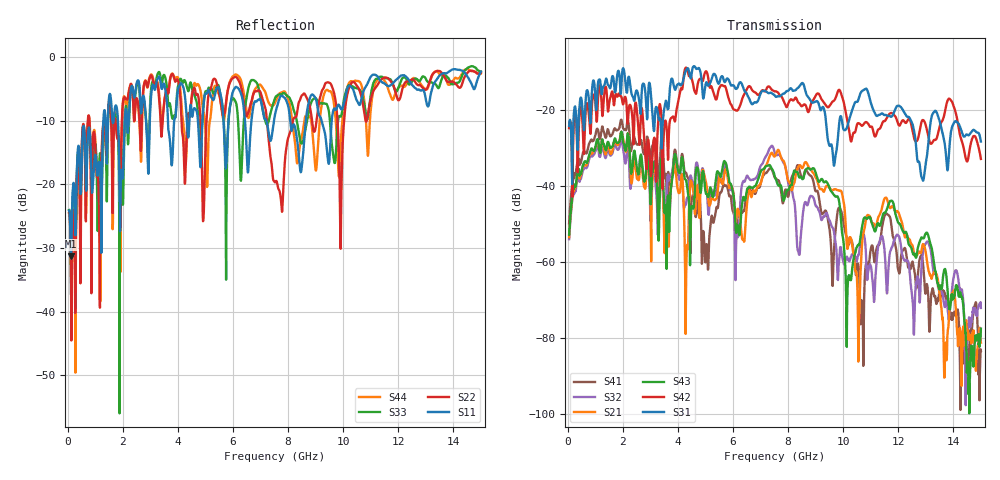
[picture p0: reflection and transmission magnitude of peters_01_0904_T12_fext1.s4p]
# MHZ S RI R 50.00
! FREQ  S11  S12  S13  S14
!  S21  S22  S23  S24
!  S31  S32  S33  S34
!  S41  S42  S43  S44
!  REAL  IMAG  REAL  IMAG  REAL  IMAG  REAL  IMAG
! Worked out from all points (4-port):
!   1496 points, 50 MHz to 15 GHz, reference 50 ohm
!   strongest paths, dB at 50 MHz, 3.79 GHz, 7.53 GHz, 11.27 GHz, 15 GHz:
!     S31: -24.2, -11.8, -16.3, -21.4, -28.3
!     S42: -24.8, -21.9, -15.1, -25.2, -32.9
!     S43: -52.8, -38.3, -37.8, -49.8, -77.5
!     S21: -53.5, -37.5, -32.0, -48.3, -81.2
!     S32: -54.0, -36.2, -31.6, -55.9, -72.1
!     S41: -49.8, -37.1, -37.9, -55.6, -83.4
!   lowest |S11| = -31.3 dB at 120 MHz (marker M1), VSWR 1.06, Z = 52.8 + j0.23 ohm
!   |S11| at or under -10 dB: start of sweep to 1.292 GHz; 8.077 GHz to 8.645 GHz (568.3 MHz wide, 6.8 % of centre); 9.215 GHz to 9.586 GHz (370.9 MHz wide, 3.95 % of centre)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
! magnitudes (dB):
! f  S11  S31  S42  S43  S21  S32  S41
! 50 MHz  -24.1  -24.2  -24.8  -52.8  -53.5  -54.0  -49.8
! 120 MHz  -31.3  -25.4  -25.0  -45.6  -46.1  -46.9  -42.6
! 3.02 GHz  -6.5  -15.9  -37.4  -44.4  -52.4  -46.0  -32.6
! 5.04 GHz  -5.8  -12.7  -9.9  -42.1  -39.8  -41.2  -55.3
! 7.64 GHz  -7.2  -16.4  -15.4  -39.8  -30.5  -31.7  -38.5
! 8.38 GHz  -15.1  -14.0  -18.1  -37.3  -34.9  -57.6  -35.0
! 15 GHz  -2.3  -28.3  -32.9  -77.5  -81.2  -72.1  -83.4
